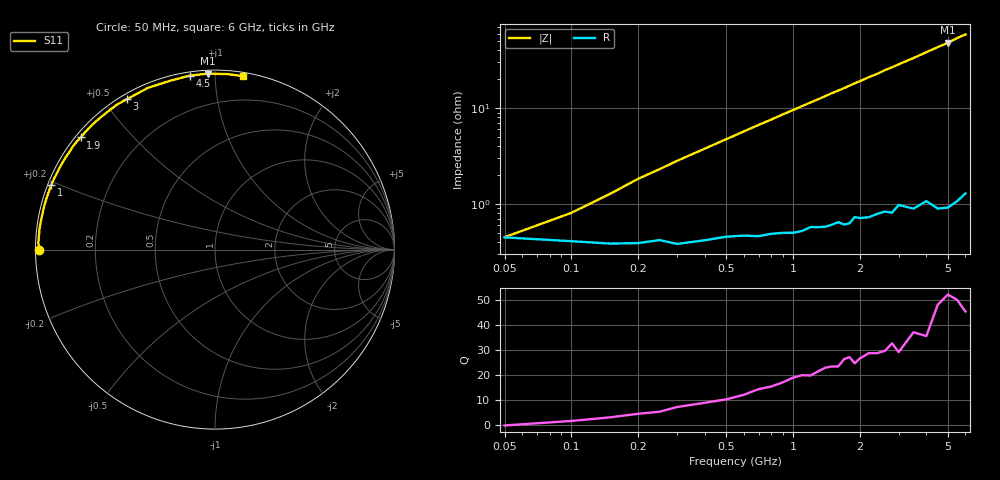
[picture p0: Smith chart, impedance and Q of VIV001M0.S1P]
! Infineon Technologies  Discrete & RF Semiconductors
! BB 804
! Si Tuning Diode in SOT23
! VR =
! S-Parameters:  July  1999
# GHz  S  MA  R  50
!  f  S11
! GHz  MAG  ANG
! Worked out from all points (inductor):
!   34 points, 50 MHz to 6 GHz, reference 50 ohm
!   read as one part to ground: L = 1.42 nH near 150 MHz
!   highest Q = 50.2 at 5 GHz (marker M1), where L = 1.53 nH
!   S11 on the Smith chart (normalised r, x): 50 MHz: 0.01, -0.00; 1 GHz: 0.01, +0.19; 1.9 GHz: 0.01, +0.36; 3 GHz: 0.02, +0.57; 4.5 GHz: 0.02, +0.86; 6 GHz: 0.03, +1.17
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0.05  0.9822 -179.9
0.1  0.9837 178.4
0.2  0.9845 175.9
0.3  0.9848 173.6
0.4  0.9835 171.4
0.6  0.9817 167.0
0.7  0.982 164.8
0.8  0.981 162.7
1  0.9808 158.4
1.2  0.9784 154.2
1.3  0.9786 152.2
1.5  0.9777 148.0
1.6  0.9765 146.1
1.7  0.9781 144.2
1.8  0.9777 142.1
1.9  0.9744 140.1
2  0.9754 138.3
2.2  0.9755 134.4
2.4  0.9742 131.0
2.6  0.9735 127.1
2.8  0.975 123.9
3  0.9709 120.4
3.5  0.9755 112.6
4  0.9733 105.1
4.5  0.9797 98.3
5  0.9811 92.3
5.5  0.9803 85.9
6  0.9785 80.9
